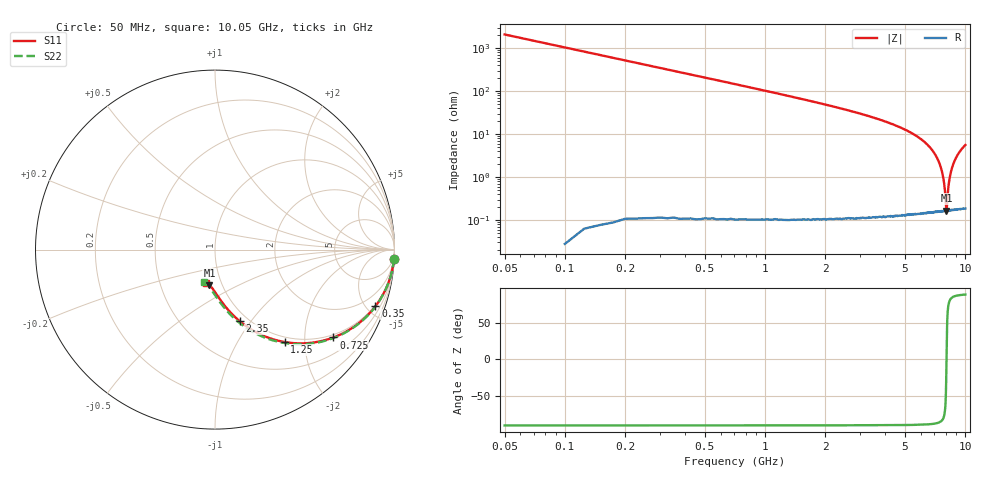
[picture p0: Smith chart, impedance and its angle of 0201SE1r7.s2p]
! AVX Thin Film Operation		Date: August 2001
! Description: Accu-P® Series, Thin Film, SMD, RF Capacitor
! Part Number: 02013J1R7ABW
! 50 MHz  -  10.05 GHz
! Serial Measurements
# mhz S db R 50
!	S11		S21		S12		S22
!	dB	Phase	dB	Phase	dB	Phase	dB	Phase
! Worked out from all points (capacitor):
!   401 points, 50 MHz to 10.05 GHz, reference 50 ohm
!   read as one part in series: C = 1.53 pF near 100 MHz
!   lowest |Z| = 166 mohm at 8.075 GHz (marker M1)
!   series resonance near 8.084 GHz, so ESL is about 250 pH
!   S11 on the Smith chart (normalised r, x): 50 MHz: 1, -40; 350 MHz: 0.92, -5.69; 725 MHz: 0.91, -2.75; 1.25 GHz: 0.91, -1.61; 2.35 GHz: 0.91, -0.88; 10.05 GHz: 0.85, -0.33
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50  -0.01 -2.9  -26.38 87.1  -26.38 87.1  -0.01 -2.9
75  -0.02 -4.3  -22.87 85.7  -22.87 85.7  -0.02 -4.4
125  -0.06 -7.2  -18.48 82.8  -18.48 82.8  -0.06 -7.2
175  -0.12 -10.0  -15.61 80.0  -15.61 80.0  -0.12 -10.1
250  -0.24 -14.1  -12.64 75.8  -12.64 75.8  -0.24 -14.3
350  -0.47 -19.5  -9.94 70.4  -9.94 70.4  -0.47 -19.7
425  -0.67 -23.3  -8.46 66.6  -8.46 66.6  -0.67 -23.5
525  -0.98 -28.1  -6.95 61.8  -6.95 61.8  -0.98 -28.3
725  -1.71 -36.6  -4.89 53.2  -4.89 53.2  -1.71 -37.0
950  -2.60 -44.6  -3.47 45.1  -3.47 45.1  -2.60 -45.1
1250  -3.81 -53.0  -2.34 36.6  -2.34 36.6  -3.81 -53.7
1475  -4.68 -58.0  -1.82 31.5  -1.82 31.5  -4.67 -58.8
1725  -5.57 -62.6  -1.42 26.8  -1.42 26.8  -5.57 -63.5
2025  -6.56 -67.1  -1.09 22.3  -1.09 22.3  -6.56 -68.2
2350  -7.51 -71.0  -0.86 18.2  -0.86 18.2  -7.51 -72.3
2825  -8.70 -75.6  -0.64 13.5  -0.64 13.5  -8.70 -77.1
3400  -9.89 -79.9  -0.48 9.0  -0.48 9.0  -9.90 -81.8
5050  -12.20 -88.6  -0.28 -0.2  -0.28 -0.2  -12.21 -91.2
6725  -13.45 -94.8  -0.21 -6.9  -0.21 -6.9  -13.47 -98.2
8075  -13.99 -99.0  -0.19 -11.5  -0.19 -11.5  -14.01 -103.1
8400  -14.08 -99.9  -0.19 -12.5  -0.19 -12.5  -14.10 -104.2
10050  -14.32 -104.5  -0.18 -17.6  -0.18 -17.6  -14.35 -109.5
